(* Logix 5000 AddOnInstructionDefinition export AKD_Command_Assembly; software revision 20.03 *)

TYPE AKD_Status :   // All connections to the drive ethernet module are established and data is successfully transferring.
STRUCT
   Profile_In_Progress : BOOL;   // Profile Move In Progress
   Block_In_Execution : BOOL;   // Block In Execution
   On_Target_Position : BOOL;   // On Target Position (1=Current Position Equals Last Target Position)
   General_Fault : BOOL;   // General Fault
   Current_Direction : BOOL;   // Current Motor Direction (0=Reverse, 1=Forward)
   Home_Level : BOOL;   // Level of Home Input
   Reg_Level : BOOL;   // Level of Registration Input
   Enable : BOOL;   // State of Enable Output
   Fault_Input_Fault : BOOL;   // Fault Input Active
   Fwd_Limit : BOOL;   // Forward Input Active
   Rev_Limit : BOOL;   // Reverse Input Active
   Positive_Limit : BOOL;   // Positive Software Limit Exceeded
   Negative_Limit : BOOL;   // Negative Software Limit Exceeded
   FE_Fault : BOOL;   // Following Error Fault
   Block_Fault : BOOL;   // Block Execution Fault
   Load_Complete : BOOL;   // Command Message Successfully Loaded
END_STRUCT
END_TYPE

TYPE AKD_Control :   // Send Explicit Message
STRUCT
   Load_Data_Start_Profile : BOOL;   // Load Command Data / Start Profile Move
   Start_Block : BOOL;   // Execute Command block or block chain
   Incremental : BOOL;   // Incremental Position (0=Absolute, 1=Incremental)
   Direction : BOOL;   // Direction in Velocity Mode (0=Reverse, 1=Forward)
   Smooth_Stop : BOOL;   // Smooth / Controlled Stop w/ Deceleration
   Hard_Stop : BOOL;   // Hard / Immediate Stop
   Reg_Arm : BOOL;   // Arm the Registration Input
   Enable : BOOL;   // Enable Output
END_STRUCT
END_TYPE

TYPE AKD_Axis :   // Axis Data:
STRUCT
   Control : AKD_Control;   // Control bits to send to the drive
   Status : AKD_Status;   // Status bits received from the drive
   Input : AB:ETHERNET_MODULE_SINT_64Bytes:I:0;   // Data from the drive
   Output : AB:ETHERNET_MODULE_SINT_64Bytes:O:0;   // Data to the drive
   ResponseMsgType : SINT;   // Response type contained in latest IO response from drive. Used to check for errors
   CommandTimeout : INT;   // Time to allow for command response from drive. Dependent on scan rate and communicaiton rate
   PositionFeedback : DINT;   // Actual Position Value
   VelocityFeedback : DINT;   // Actual Velocity Value
END_STRUCT
END_TYPE

ADD_ON_INSTRUCTION AKD_Command_Assembly   (* revision 2.0 *)
// Revision note:
// Output Data Bytes 12-15 changed to velocity tag
// ( was position; a duplicate ).
VAR_IN_OUT
   Axis : AKD_Axis; {required}
END_VAR
VAR_OUTPUT
   Control_Word : SINT; {access Read Only, visible}
   Block_Number : SINT; {access Read Only, visible}
   Command_Type : SINT; {access Read Only, visible}
   Response_Type : SINT; {access Read Only, visible}
   Data : DINT; {access Read Only, visible}
   Position : DINT; {access Read Only, visible}
   Velocity : DINT; {access Read Only, visible}
   Acceleration : DINT; {access Read Only, visible}
   Deceleration : DINT; {access Read Only, visible}
   Parameter_Attribute_Data : DINT; {access Read Only, visible}
   Attribute_To_Get : DINT; {access Read Only, visible}
   Map_Type : SINT; {access Read Only, visible}
END_VAR

ROUTINE Logic   (* ladder *)
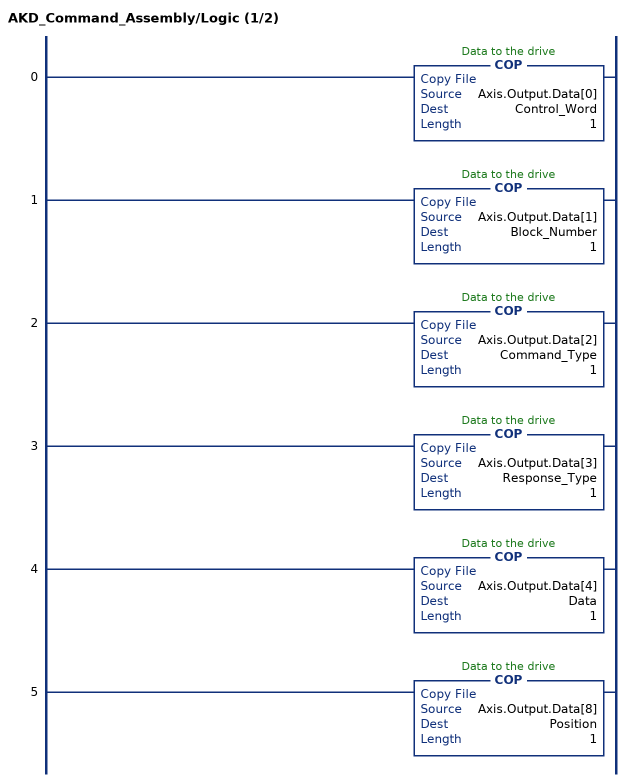
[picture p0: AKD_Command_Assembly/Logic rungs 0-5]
   0: COP(Axis.Output.Data[0],Control_Word,1);
   1: COP(Axis.Output.Data[1],Block_Number,1);
   2: COP(Axis.Output.Data[2],Command_Type,1);
   3: COP(Axis.Output.Data[3],Response_Type,1);
   4: COP(Axis.Output.Data[4],Data,1);
   5: COP(Axis.Output.Data[8],Position,1);
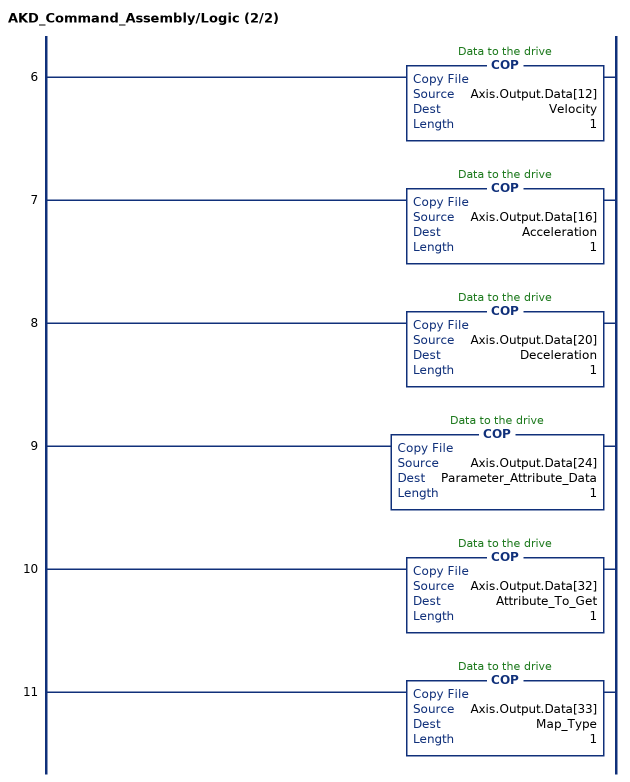
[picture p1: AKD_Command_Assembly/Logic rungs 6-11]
   6: COP(Axis.Output.Data[12],Velocity,1);
   7: COP(Axis.Output.Data[16],Acceleration,1);
   8: COP(Axis.Output.Data[20],Deceleration,1);
   9: COP(Axis.Output.Data[24],Parameter_Attribute_Data,1);
   10: COP(Axis.Output.Data[32],Attribute_To_Get,1);
   11: COP(Axis.Output.Data[33],Map_Type,1);
END_ROUTINE
END_ADD_ON_INSTRUCTION
